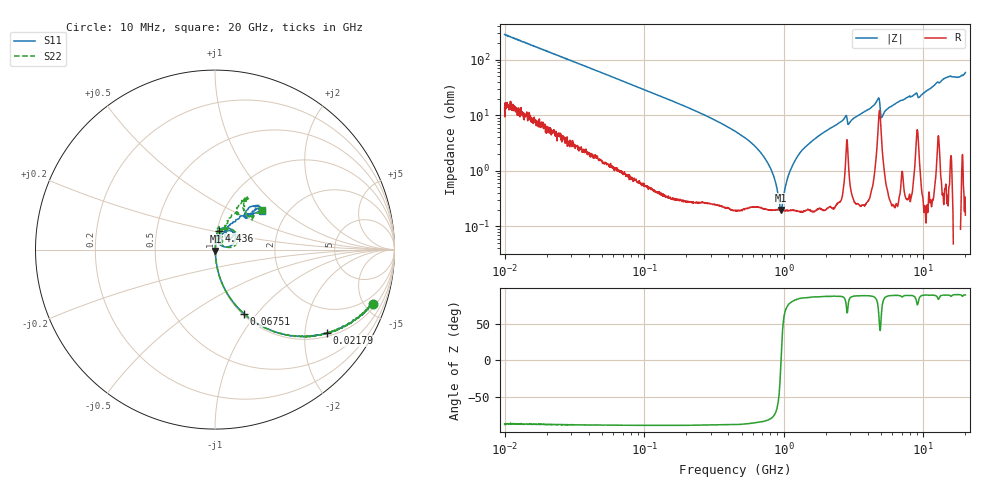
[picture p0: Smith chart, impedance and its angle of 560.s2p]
!Keysight Technologies,P5008B,MY61100088,A.16.20.02
!Date: Friday, August 30, 2024 14:18:49
!Correction: S11(C  2-Port  )
!S21(C  2-Port  )
!S12(C  2-Port  )
!S22(C  2-Port  )
!S2P File: Measurements: S11, S21, S12, S22:Log Frequency Sweep
# Hz S  MA  R 50
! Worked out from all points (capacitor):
!   1601 points, 10 MHz to 20 GHz, reference 50 ohm
!   read as one part in series: C = 55.9 pF near 10.39 MHz
!   lowest |Z| = 196 mohm at 956.4 MHz (marker M1)
!   series resonance near 955.3 MHz, so ESL is about 500 pH
!   S11 on the Smith chart (normalised r, x): 10 MHz: 1.26, -5.69; 21.79 MHz: 1.11, -2.60; 67.51 MHz: 1.02, -0.86; 4.436 GHz: 1.02, +0.22; 20 GHz: 1.49, +0.73
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1e7  0.9305 -19.1  0.3267 68.2  0.3267 68.3  0.9299 -19.1
2.179493e7  0.778 -36.7  0.5976 51.0  0.5974 51.0  0.7778 -36.7
3.555162e7  0.6214 -49.9  0.7648 38.4  0.7647 38.4  0.6213 -49.9
6.751244e7  0.3914 -65.7  0.9113 23.0  0.9111 23.0  0.3913 -65.7
1.263918e8  0.2233 -76.2  0.9708 12.8  0.9707 12.8  0.2233 -76.4
4.472136e8  0.05538 -84.9  0.9964 2.7  0.996 2.7  0.0553 -86.2
7.470239e8  0.02147 -83.5  0.9976 0.5  0.9974 0.5  0.02142 -86.1
9.563525e8  0.008151 -72.2  0.9978 -0.4  0.9977 -0.5  0.007744 -84.2
1.012455e9  0.004943 -59.7  0.9979 -0.7  0.9977 -0.7  0.004212 -80.8
1.061713e9  0.003266 -26.8  0.9979 -0.9  0.9978 -0.9  0.001446 -72.7
1.092411e9  0.003332 1.2  0.998 -1.0  0.9978 -1.0  0.0002302 56.4
1.173095e9  0.005756 45.1  0.9981 -1.3  0.9978 -1.3  0.004047 92.7
1.253768e9  0.009094 68.2  0.9981 -1.6  0.9978 -1.6  0.00835 87.2
1.589917e9  0.0216 80.8  0.9979 -2.7  0.9976 -2.7  0.02121 84.9
4.436224e9  0.1064 78.0  0.9868 -11.2  0.9865 -11.2  0.1063 71.4
4.71883e9  0.1398 60.7  0.9464 -13.2  0.9464 -13.3  0.1423 56.0
5.140092e9  0.04397 65.9  0.9839 -9.0  0.9838 -9.0  0.04782 53.8
5.652411e9  0.07037 76.1  0.9954 -11.5  0.9951 -11.6  0.07315 74.1
7.697294e9  0.1229 61.8  0.9926 -17.2  0.9923 -17.4  0.1204 78.9
9.486728e9  0.09455 54.6  0.9894 -20.0  0.9892 -20.2  0.08924 70.1
1.44103e10  0.3238 47.8  0.9516 -34.4  0.9512 -34.6  0.3166 59.9
2e10  0.3386 39.8  0.9418 -49.7  0.9418 -50.0  0.3411 40.2
